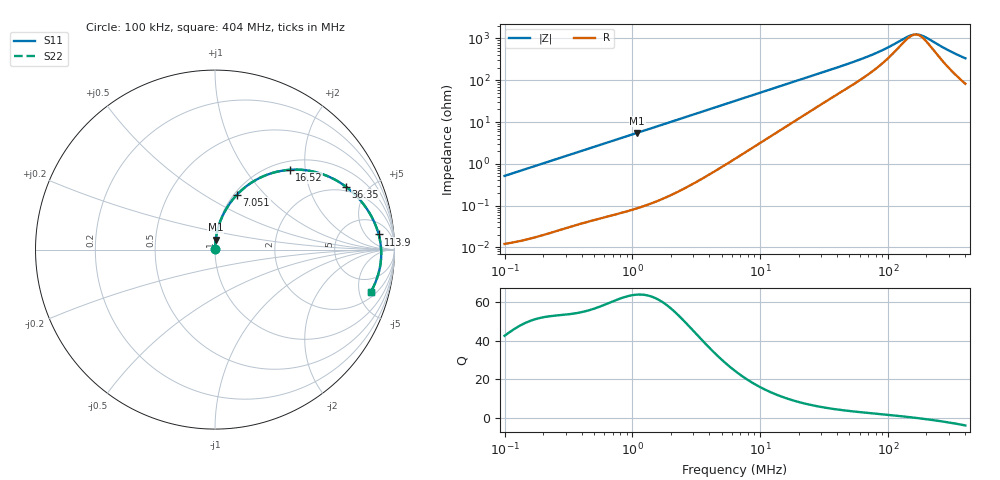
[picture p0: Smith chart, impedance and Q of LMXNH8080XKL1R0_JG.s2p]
! LMXNH8080XKL1R0_JG  S-PARAMETER MODEL  ( General Type )
! Model Generated by TAIYO YUDEN Corporation (http://www.ty-top.com)
! Version 1.0
! TAIYO YUDEN Control No. 191025NI43SB-FBB
! Copyright(c) 2019 TAIYO YUDEN CO.,LTD. All Rights Reserved.
! Product Description (link to TY-COMPAS)
! https://ds.yuden.co.jp/TYCOMPAS/or/detail?pn=LMXNH8080XKL1R0NJG&u=M
! Products Name : Inductors
! Characteristics :
!  Inductance : 1.0 uH , SRF(min) : 120 MHz , DC Resistance(max) : 0.0117 Ohm
!  Rated Current : Saturation :7800 mA , Temp Rise : 6200 mA
!  Case Size : 8.0 x 8.0 / 0.315 x 0.315 [mm/inch] , Thickness : 3 / 0.118 [mm/inch]
!  (Conditions: Temperature = 25 degC , DC Bias Current/Voltage = 0A / 0V)
! External Node Assignments :
!  1  o---GGG---o  2
! GND o---------o GND
! Frequency Range : 0.1MHz  -  403.964729MHz  [ 402 STEP ]
# MHz S RI R 50
! Freq[MHz].  S11 Real  S11 Imag  S21 Real  S21 Imag  S12 Real  S12 Imag  S22 Real  S22 Imag
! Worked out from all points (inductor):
!   401 points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, 100 kHz to 404 MHz, reference 50 ohm
!   read as one part in series: L = 818 nH near 104.2 kHz
!   highest Q = 63.7 at 1.088 MHz (marker M1), where L = 804 nH
!   self-resonance near 163.7 MHz
!   S11 on the Smith chart (normalised r, x): 100 kHz: 1.00, +0.01; 7.051 MHz: 1.03, +0.71; 16.52 MHz: 1.17, +1.65; 36.35 MHz: 1.76, +3.57; 113.9 MHz: 11, +11; 404 MHz: 2.64, -6.50
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0.1  0.000148 0.00514  0.9999 -0.00514  0.9999 -0.00514  0.000148 0.00514
0.401849  0.000792 0.0204  0.9992 -0.0204  0.9992 -0.0204  0.000792 0.0204
1.088488  0.00386 0.0547  0.9961 -0.0547  0.9961 -0.0547  0.00386 0.0547
1.614823  0.00789 0.0807  0.9921 -0.0807  0.9921 -0.0807  0.00789 0.0807
3.628637  0.0365 0.1752  0.9635 -0.1752  0.9635 -0.1752  0.0365 0.1752
6.355822  0.1024 0.2832  0.8976 -0.2832  0.8976 -0.2832  0.1024 0.2832
7.051005  0.1227 0.3062  0.8773 -0.3062  0.8773 -0.3062  0.1227 0.3062
10.4605  0.2314 0.3901  0.7686 -0.3901  0.7686 -0.3901  0.2314 0.3901
16.51586  0.4161 0.4446  0.5839 -0.4446  0.5839 -0.4446  0.4161 0.4446
25.54079  0.6058 0.4178  0.3942 -0.4178  0.3942 -0.4178  0.6058 0.4178
36.34995  0.7292 0.3506  0.2708 -0.3506  0.2708 -0.3506  0.7292 0.3506
47.6113  0.7982 0.2879  0.2018 -0.2879  0.2018 -0.2879  0.7982 0.2879
65.00517  0.8547 0.2138  0.1453 -0.2138  0.1453 -0.2138  0.8547 0.2138
83.39465  0.8862 0.1557  0.1138 -0.1557  0.1138 -0.1557  0.8862 0.1557
102.6353  0.905 0.108  0.095 -0.108  0.095 -0.108  0.905 0.108
113.8613  0.9121 0.0842  0.0879 -0.0842  0.0879 -0.0842  0.9121 0.0842
149.1359  0.9238 0.0219  0.0762 -0.0219  0.0762 -0.0219  0.9238 0.0219
162.0487  0.9255 0.00245  0.0745 -0.00245  0.0745 -0.00245  0.9255 0.00245
176.0796  0.9262 -0.0172  0.0738 0.0172  0.0738 0.0172  0.9262 -0.0172
199.4363  0.9254 -0.0472  0.0746 0.0472  0.0746 0.0472  0.9254 -0.0472
308.4163  0.9028 -0.159  0.0972 0.159  0.0972 0.159  0.9028 -0.159
403.9647  0.8687 -0.2342  0.1313 0.2342  0.1313 0.2342  0.8687 -0.2342
